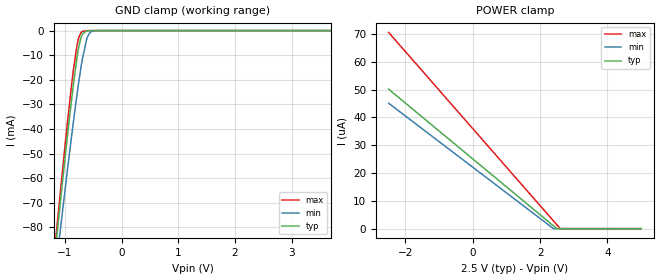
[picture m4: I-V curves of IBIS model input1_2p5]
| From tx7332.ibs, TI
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|   input1_2p5 Model
[Model]   input1_2p5
Model_type   Input
Vinl = 0.625
Vinh = 1.875
|   typ   min   max
C_comp   2.990pF   2.962pF   3.032pF
[Model spec]
|subparameter
Vinl   0.625   0.6   0.65
Vinh   1.875   1.8   1.95
| Where Nom  PVT is Nominal Process, 2.5V, 27C
|   Fast PVT is Strong Process,  2.6V, 0C
|   Slow PVT is Weak Process,   2.4V, 100C
[Voltage Range]   2.5   2.4   2.6
|Junction Temperature
[Temperature Range]   27   100   0
[Power Clamp Reference]   2.5   2.4   2.6
[GND Clamp Reference]   0   0   0
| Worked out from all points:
|   GND clamp passes 1 mA (typ) near -0.67 V on its own axis
[GND Clamp]
|   Voltage   I(typ)   I(min)   I(max)
-2.5V     -400.5mA   -375.1mA   -414.6mA
-1.173V   -90.46mA   -99.43mA   -87.36mA
-1.075V   -68.76mA   -80.04mA   -64.5mA
-955mV    -42.91mA   -56.73mA   -37.42mA
-850mV    -21.96mA   -37.2mA    -16.04mA
-767.5mV  -8.348mA   -22.94mA   -3.922mA
-722.5mV  -3.377mA   -15.91mA   -1.027mA
-692.5mV  -1.486mA   -11.68mA   -357.9uA
-595mV    -55.46uA   -2.339mA   -19.83uA
-542.5mV  -12.55uA   -625.3uA   -9.657uA
-467.5mV  -5.101uA   -75.7uA    -6.633uA
5V        0A         0A         0A
[POWER Clamp]
|   Voltage   I(typ)   I(min)   I(max)
-2.5V     50.19uA    45.13uA    70.6uA
2.39V     1.073uA    57.87nA    2.877uA
2.495V    17.36nA    0A         1.422uA
2.592V    0A         0A         71.53nA
5V        0A         0A         0A
